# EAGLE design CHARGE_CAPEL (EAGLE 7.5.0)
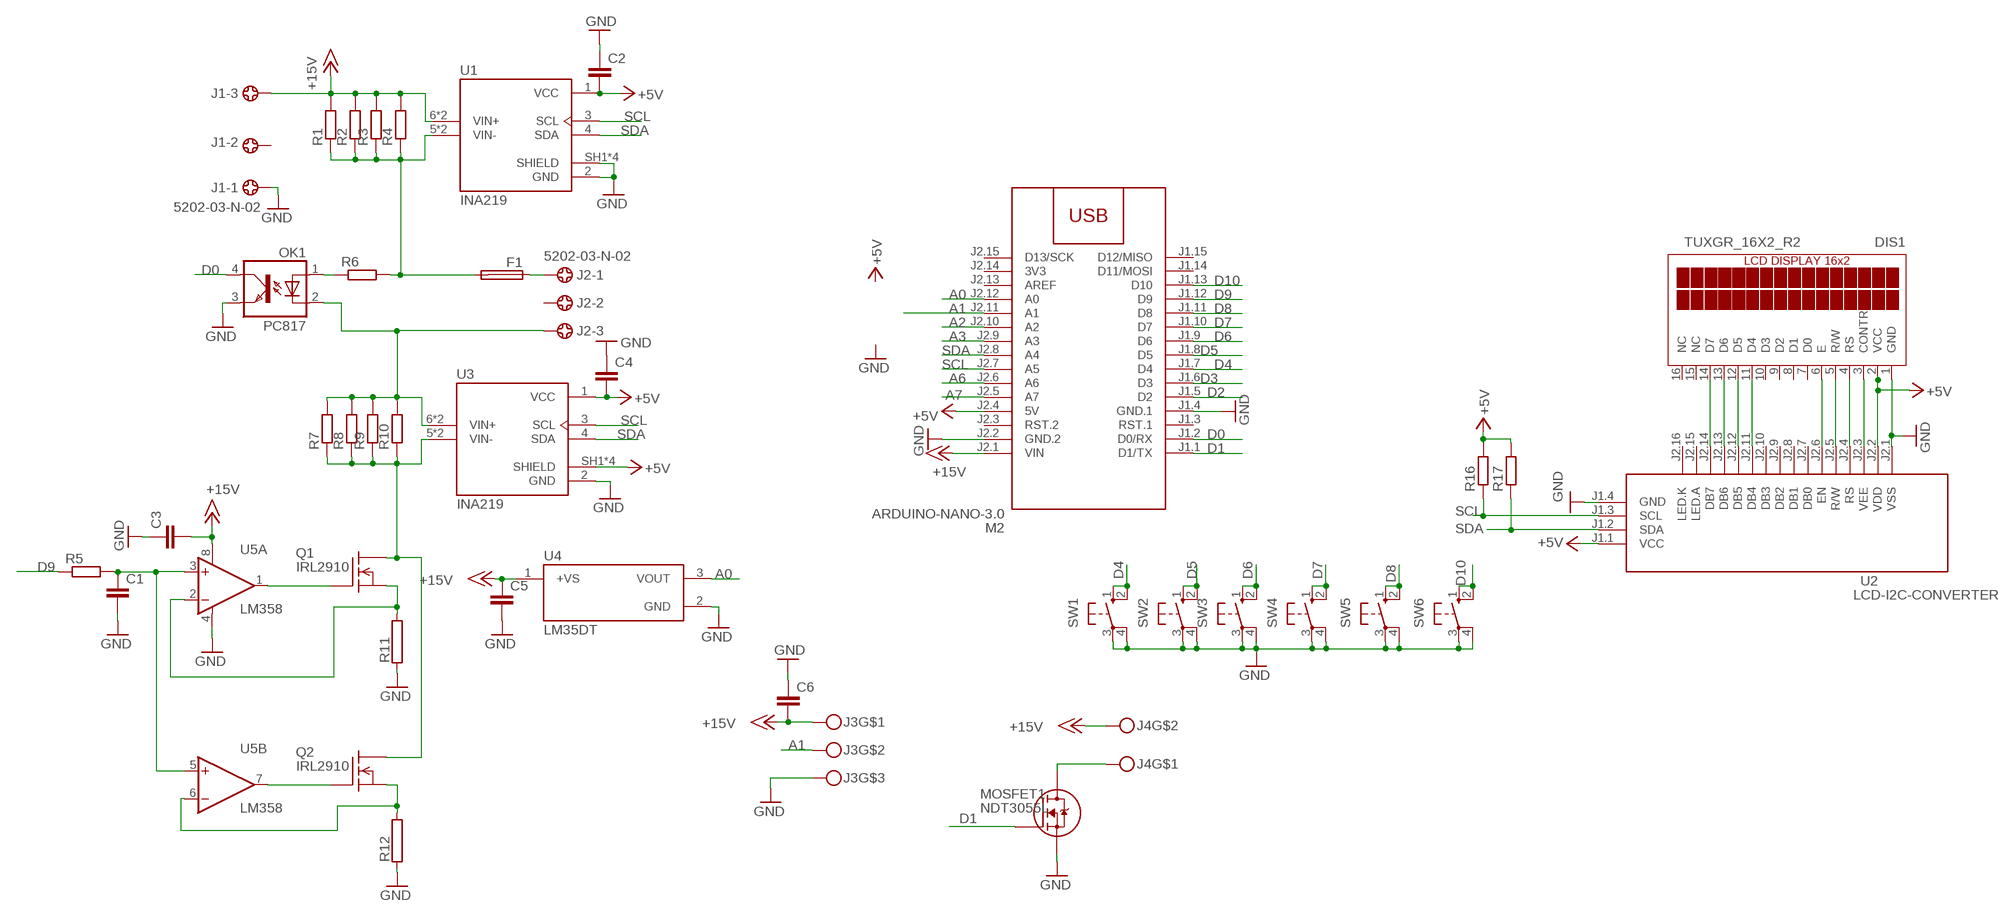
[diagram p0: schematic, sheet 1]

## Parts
C1  C-EUC1206  [C1206]
C2  C-EUC1206  [C1206]
C3  C-EUC1206  [C1206]
C4  C-EUC1206  [C1206]
C5  C-EUC1206  [C1206]
C6  C-EUC1206  [C1206]
DIS1  TUXGR_16X2_R2  [TUXGR_16X2_R2]
F1  FUSEBLANK_5X20MM  [FUSE_HOLDER_5X20MM]
J1  5202-03-N-02  [5202-03-N-02]
J2  5202-03-N-02  [5202-03-N-02]
J3  MKDSN3  [MKDSN3]
J4  MKDSN1,5-2-5,08  [MKDSN1,5-2-5,08]
M2  ARDUINO-NANO-3.0  [ARDUINO-NANO-3.0]
MOSFET1  NDT3055L  [SOT223-4]
OK1  PC817  [DIL04]
Q1  IRL2910  IRF540  [TO220]
Q2  IRL2910  IRF540  [TO220]
R1  R-EU_R2512  [R2512]
R2  R-EU_R2512  [R2512]
R3  R-EU_R2512  [R2512]
R4  R-EU_R2512  [R2512]
R5  R-EU_R1206  [R1206]
R6  R-EU_R1206  [R1206]
R7  R-EU_R2512  [R2512]
R8  R-EU_R2512  [R2512]
R9  R-EU_R2512  [R2512]
R10  R-EU_R2512  [R2512]
R11  RCA4200  [CA4200]
R12  RCA4200  [CA4200]
R16  R-EU_R1206  [R1206]
R17  R-EU_R1206  [R1206]
SW1  40-XX  [B3F-40XX]
SW2  40-XX  [B3F-40XX]
SW3  40-XX  [B3F-40XX]
SW4  40-XX  [B3F-40XX]
SW5  40-XX  [B3F-40XX]
SW6  40-XX  [B3F-40XX]
U1  INA219  [MODULE_INA219]
U2  LCD-I2C-CONVERTER  [LCD-I2C-CONVERTER]
U3  INA219  [MODULE_INA219]
U4  LM35DT  [TO254P1016X457X1955-3]
U5  LM358  OPA2234P  [DIL08]

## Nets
+5V: C2.2 C4.2 DIS1.2(VCC) M2.J2.4(5V) R16.2 R17.2 U1.1(VCC) U2.J1.1(VCC) U2.J2.2(VDD) U3.1(VCC) U3.SH1(SHIELD) U3.SH2(SHIELD) U3.SH3(SHIELD) U3.SH4(SHIELD)
+15V: C3.2 C5.1 C6.2 J1.3 J3.1 J4.2 M2.J2.1(VIN) R1.2 R2.2 R3.2 R4.2 U1.6(VIN+) U1.VIN+ U4.1(+VS) U5.8(A:V+)
A0: M2.J2.12(A0) U4.3(VOUT)
A1: J3.2 M2.J2.11(A1)
A2: M2.J2.10(A2)
A3: M2.J2.9(A3)
A6: M2.J2.6(A6)
A7: M2.J2.5(A7)
D0: M2.J1.2(D0/RX) OK1.4(COL)
D1: M2.J1.1(D1/TX) MOSFET1.1(G)
D2: M2.J1.5(D2)
D3: M2.J1.6(D3)
D4: M2.J1.7(D4) SW1.1(S) SW1.2(S1)
D5: M2.J1.8(D5) SW2.1(S) SW2.2(S1)
D6: M2.J1.9(D6) SW3.1(S) SW3.2(S1)
D7: M2.J1.10(D7) SW4.1(S) SW4.2(S1)
D8: M2.J1.11(D8) SW5.1(S) SW5.2(S1)
D9: M2.J1.12(D9) R5.1
D10: M2.J1.13(D10) SW6.1(S) SW6.2(S1)
GND: C1.2 C2.1 C3.1 C4.1 C5.2 C6.1 DIS1.1(GND) J1.1 J3.3 M2.J1.4(GND.1) M2.J2.2(GND.2) MOSFET1.3(S) OK1.3(EMIT) R11.1 R12.1 SW1.3(P) SW1.4(P1) SW2.3(P) SW2.4(P1) SW3.3(P) SW3.4(P1) SW4.3(P) SW4.4(P1) SW5.3(P) SW5.4(P1) SW6.3(P) SW6.4(P1) U1.2(GND) U1.SH1(SHIELD) U1.SH2(SHIELD) U1.SH3(SHIELD) U1.SH4(SHIELD) U2.J1.4(GND) U2.J2.1(VSS) U3.2(GND) U4.2(GND) U5.4(A:V-)
N$1: DIS1.14(D7) U2.J2.14(DB7)
N$2: DIS1.13(D6) U2.J2.13(DB6)
N$3: DIS1.12(D5) U2.J2.12(DB5)
N$4: DIS1.11(D4) U2.J2.11(DB4)
N$5: DIS1.6(E) U2.J2.6(EN)
N$6: DIS1.5(R/W) U2.J2.5(R/W)
N$7: DIS1.4(RS) U2.J2.4(RS)
N$8: Q1.1(G) U5.1(A:OUT)
N$9: F1.2 R1.1 R2.1 R3.1 R4.1 R6.2 U1.5(VIN-) U1.VIN-
N$10: DIS1.3(CONTR) U2.J2.3(VEE)
N$11: F1.1 J2.1
N$12: J2.3 OK1.2(C) R7.2 R8.2 R9.2 R10.2 U3.6(VIN+) U3.VIN+
N$13: OK1.1(A) R6.1
N$14: Q1.3(S) R11.2 U5.2(A:-IN)
N$15: Q2.3(S) R12.2 U5.6(B:-IN)
N$16: Q1.2(D) Q2.2(D) R7.1 R8.1 R9.1 R10.1 U3.5(VIN-) U3.VIN-
N$17: Q2.1(G) U5.7(B:OUT)
N$18: J4.1 MOSFET1.2(D) MOSFET1.4(D)
N$19: C1.1 R5.2 U5.3(A:+IN) U5.5(B:+IN)
SCL: M2.J2.7(A5) R16.1 U1.3(SCL) U2.J1.3(SCL) U3.3(SCL)
SDA: M2.J2.8(A4) R17.1 U1.4(SDA) U2.J1.2(SDA) U3.4(SDA)
Unconnected: DIS1.7(D0) DIS1.8(D1) DIS1.9(D2) DIS1.10(D3) DIS1.15(NC) DIS1.16(NC) J1.2 J2.2 M2.J1.3(RST.1) M2.J1.14(D11/MOSI) M2.J1.15(D12/MISO) M2.J2.3(RST.2) M2.J2.13(AREF) M2.J2.15(D13/SCK) U2.J2.7(DB0) U2.J2.8(DB1) U2.J2.9(DB2) U2.J2.10(DB3) U2.J2.15(LED.A) U2.J2.16(LED.K)

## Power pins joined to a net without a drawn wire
3V3: M2.J2.14(3V3)

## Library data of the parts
C1-C6 = rcl:C-EU: CAPACITOR, European symbol
DIS1 = display-lcd:TUXGR_16X2_R2: Tuxgraphics LCD display 16x2 characters reflective, without background light Source: tuxgr_12x2_r2.pdf; OC_FARNELL: unknown; OC_NEWARK: unknown
F1 = fuse:FUSE: Fuse; OC_FARNELL: unknown; OC_NEWARK: unknown
J1 J2 = con-ebyelectro:5202-03-N-02: Barrier Blocks Sreies 5202 Source: http://www.ebyelectro.com/PDF/5202-XX-N-02.pdf; OC_FARNELL: unknown; OC_NEWARK: unknown
J3 = con-phoenix-508:MKDSN3
J4 = con-phoenix-508:MKDSN1,5-2-5,08
M2 = diy-modules:ARDUINO-NANO-3.0: Arduino Nano 3.0 and compatible devices More details available here: https://www.arduino.cc/en/Main/ArduinoBoardNano Click here to find device on ebay.com
MOSFET1 = NDT3055L:NDT3055L: Trans MOSFET N-CH 60V 4A 4-Pin(3+Tab) SOT-223 Trans MOSFET N-CH 60V 4A 4-Pin(3+Tab) SOT-223 Check availability; AVAILABILITY: In Stock; CHECK_PRICES: https://www.snapeda.com/parts/NDT3055L/Onsemi/view-part/?ref=eda; DESCRIPTION: Trans MOSFET N-CH 60V 4A 4-Pin(3+Tab) SOT-223 Trans MOSFET N-CH 60V 4A 4-Pin(3+Tab) SOT-223; MF: ON; MP: NDT3055L; PACKAGE: SOT-223-4 Fairchild Semiconductor; PRICE: None; SNAPEDA_LINK: https://www.snapeda.com/parts/NDT3055L/Onsemi/view-part/?ref=snap
OK1 = optocoupler:PC817: SHARP OPTO COUPLER; MPN: PC817X4J000F; OC_FARNELL: 9707727; OC_NEWARK: 97K7059
Q1 Q2 = transistor-fet:IRF540: N-Channel Enhancement MOSFET (HEXFET); 100V; 28A; 0,077Ohm
R1-R10 R16 R17 = rcl:R-EU_: RESISTOR, European symbol
R11 R12 = resistor-power:R: Power Resitor; OC_FARNELL: unknown; OC_NEWARK: unknown
SW1-SW6 = switch-omron:40-XX: OMRON SWITCH; MF: OMRON COMPONENTS USA; MPN: B3F-4000; OC_FARNELL: 176434; OC_NEWARK: 36K3105
U1 U3 = INA219:INA219: Check availability; AVAILABILITY: Not in stock; CHECK_PRICES: https://www.snapeda.com/parts/INA219%20High%20Side%20DC%20Current%20Sensor%20Breakout%20-%2026V%20%C2%B13.2A%20Max%20-%20STEMMA%20QT/Adafruit+Industries/view-part/?ref=eda; DESCRIPTION: INA219 High Side DC Current Sensor Breakout - 26V ±3.2A Max | Adafruit Industries 904; MF: Adafruit Industries; MP: INA219 High Side DC Current Sensor Breakout - 26V ±3.2A Max - STEMMA QT; PACKAGE: NON-STANDARD-8 ADAFRUIT; PRICE: None; SNAPEDA_LINK: https://www.snapeda.com/parts/INA219%20High%20Side%20DC%20Current%20Sensor%20Breakout%20-%2026V%20%C2%B13.2A%20Max%20-%20STEMMA%20QT/Adafruit+Industries/view-part/?ref=snap
U2 = diy-modules:LCD-I2C-CONVERTER: I2C Bus to 4-Bit Parallel LCD Interface with LED backlight driver
U4 = LM35DT-H:LM35DT: Check availability; AVAILABILITY: In Stock; CHECK_PRICES: https://www.snapeda.com/parts/LM35DT/Texas+Instruments/view-part/?ref=eda; DESCRIPTION: ±0.5°C 4V-30V, Temperature sensor with analog output 3-TO-220 0 to 100; MF: Texas Instruments; MP: LM35DT; PACKAGE: TO-220-3 Texas Instruments; PRICE: None; SNAPEDA_LINK: https://www.snapeda.com/parts/LM35DT/Texas+Instruments/view-part/?ref=snap
U5 = burr-brown:OPA2234: Operational Amplifier; OC_FARNELL: unknown; OC_NEWARK: unknown

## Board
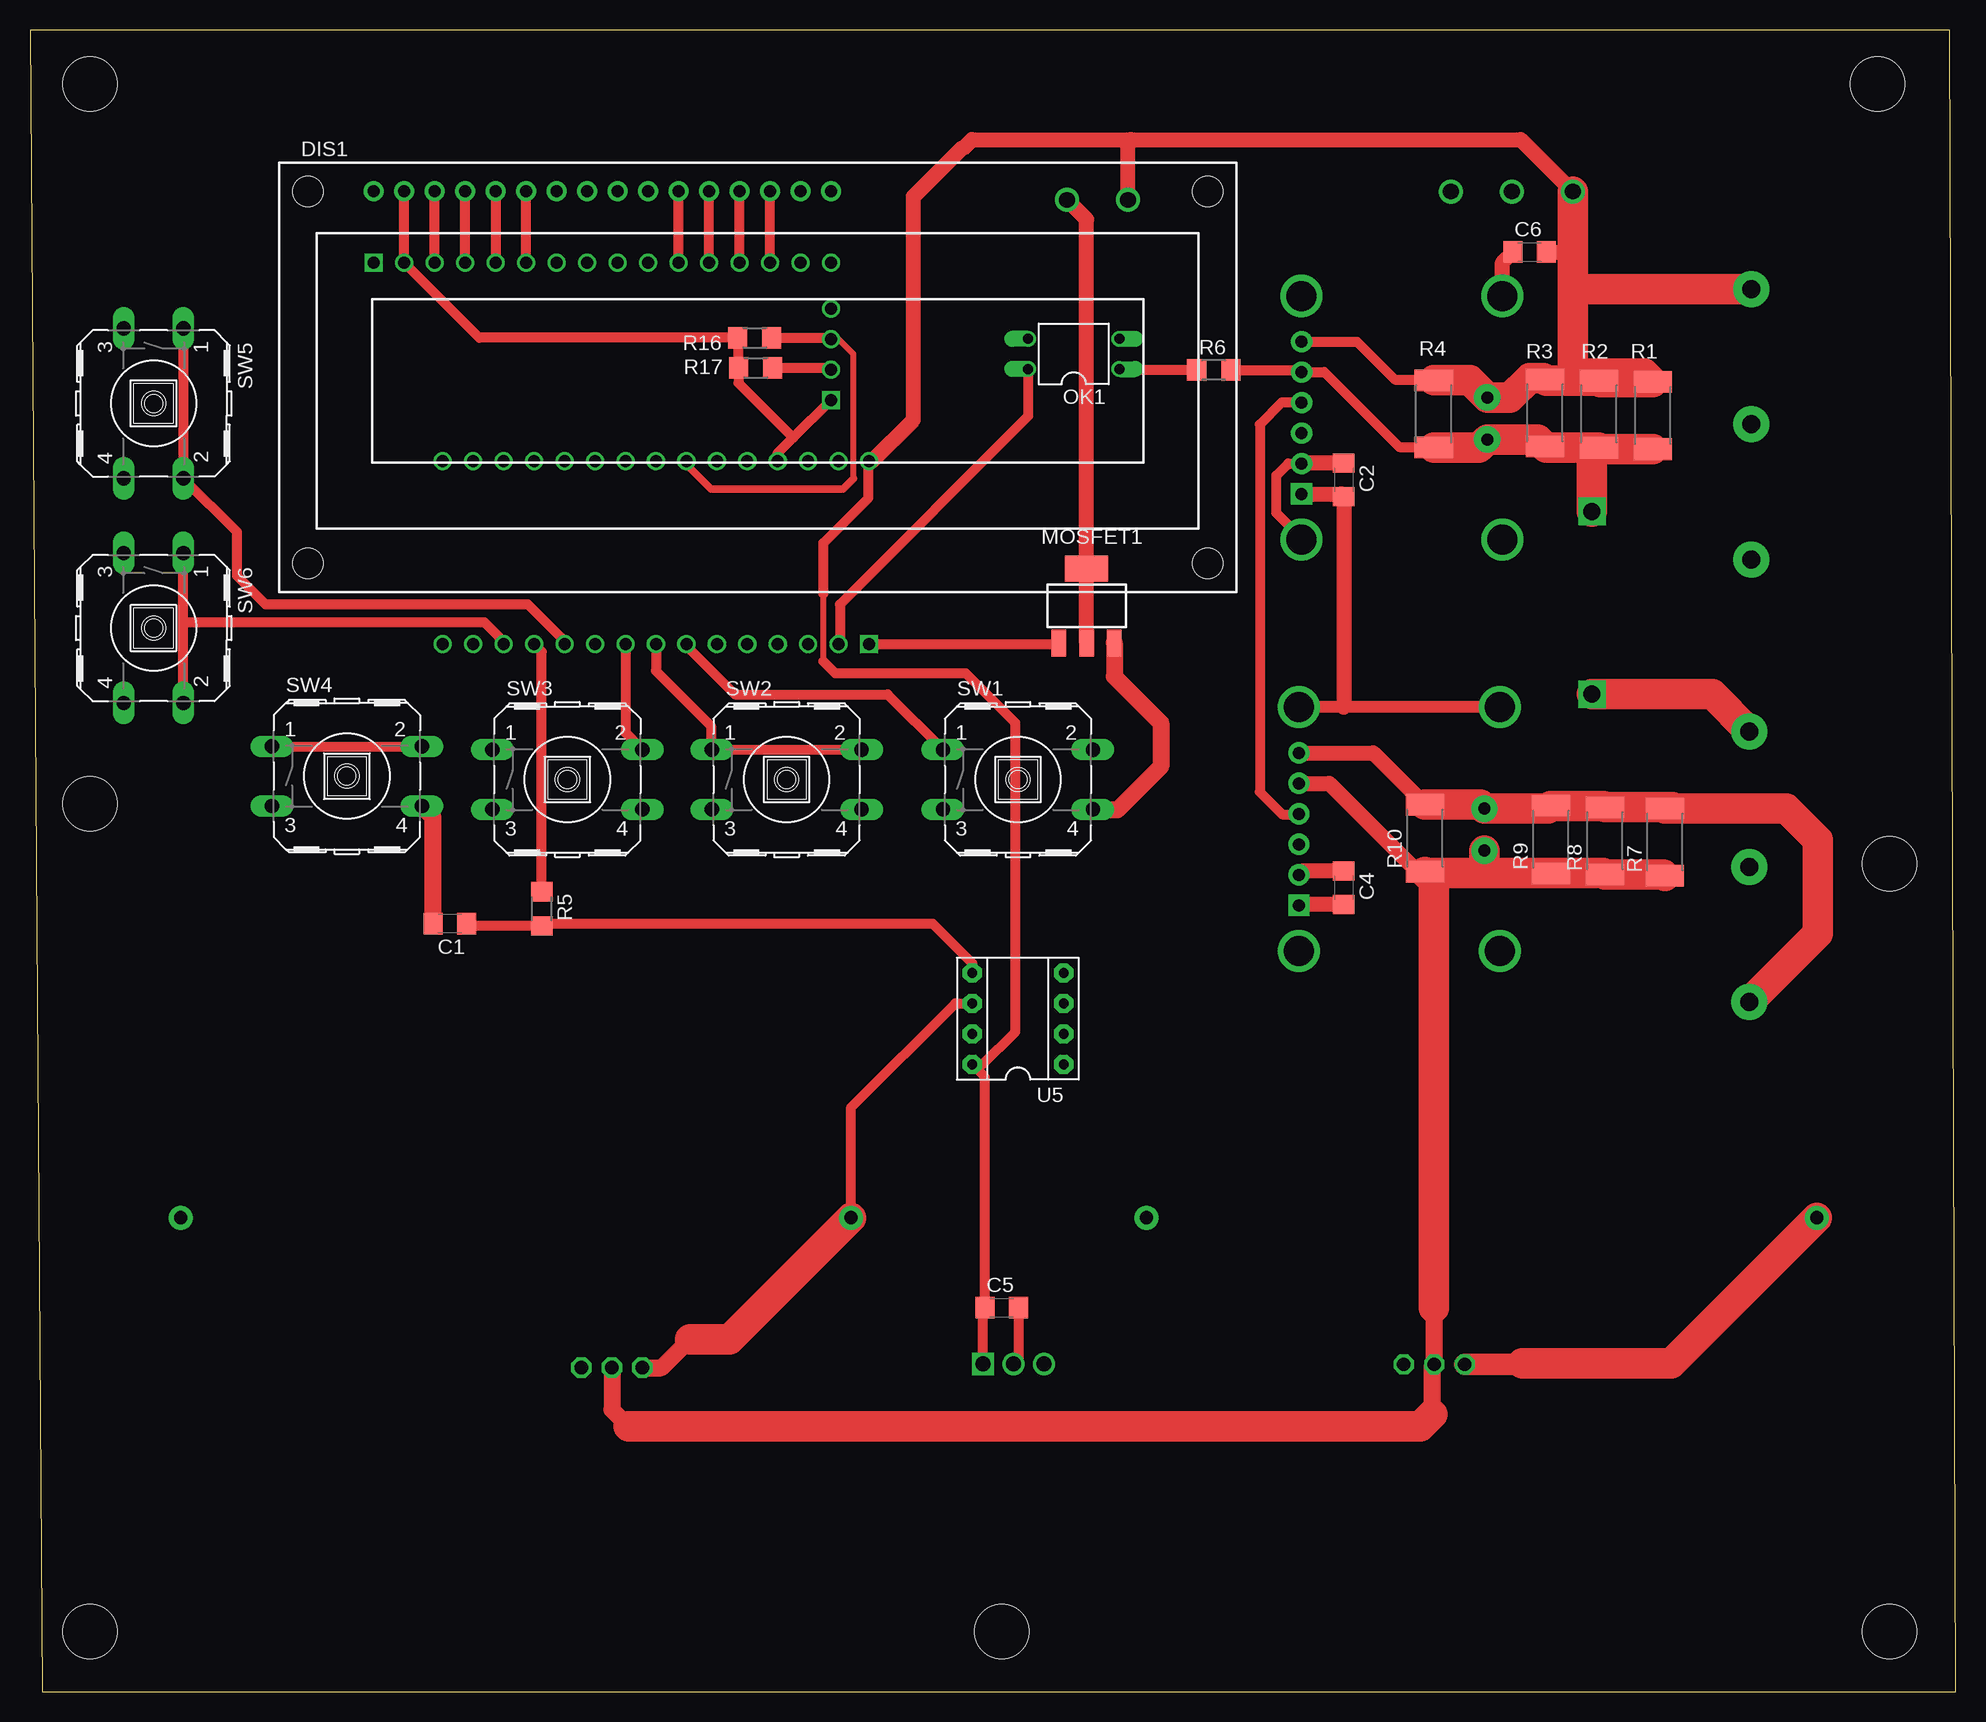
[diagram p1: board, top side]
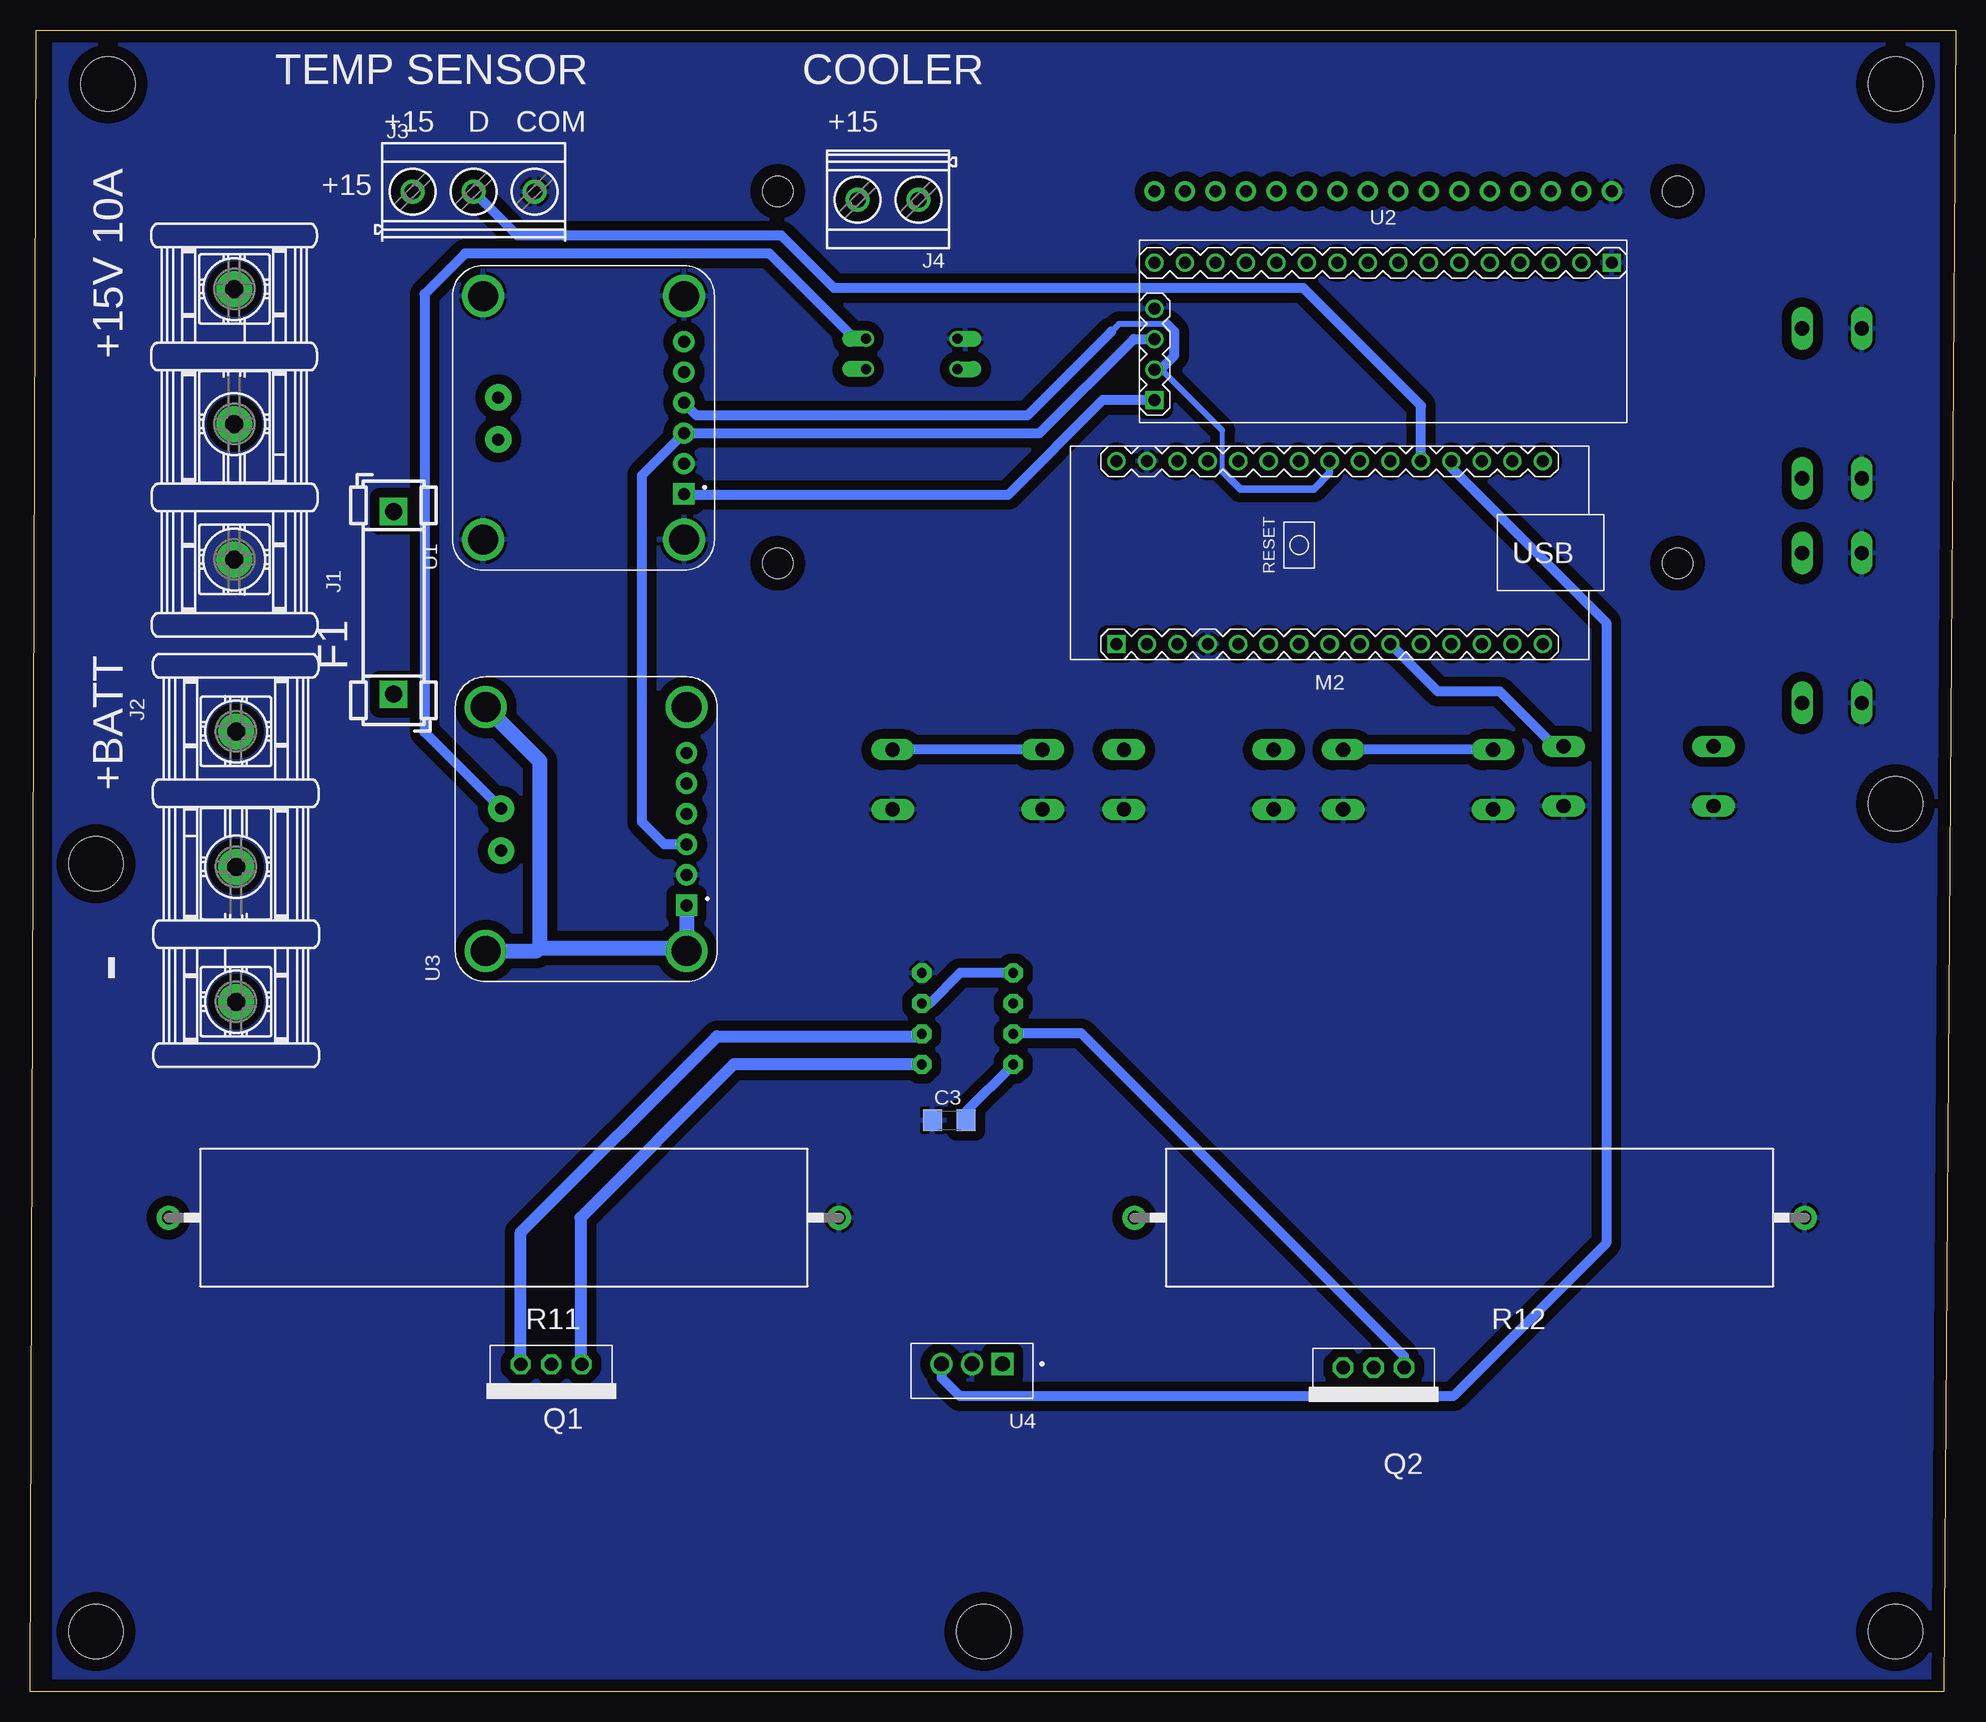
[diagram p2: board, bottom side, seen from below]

Size 160.5 x 138.5 mm. Coordinates in mm from the lower left corner, seen from the top.
Outline: 1,0 160.5,0 160,138.5 0,138.5 1,0
Copper layers (1*16): Top 0.035mm / dielectric 1.5mm / Bottom 0.035mm
Design rules "default": minimum track width 10mil, minimum drill 24mil, track to track 8mil, track to pad 8mil, pad to pad 8mil, via to via 8mil, smd to smd 8mil, copper to edge 40mil, drill to drill 8mil, minimum pad ring 10mil, minimum via ring 8mil, stop-mask expansion 4mil, vias tented up to drill 0mil, thermal gap 10mil
Holes 4.5 mm at 5,134 5,74 5,5 81,5 155,5 155,69 154,134

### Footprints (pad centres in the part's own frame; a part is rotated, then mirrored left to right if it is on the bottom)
C1206 = smd 1.6 x 1.8: 1 -1.4,0; 2 1.4,0
TUXGR_16X2_R2 = drill 1 pad 1.676: 1 -32,15.5; 2 -29.46,15.5; 3 -26.92,15.5; 4 -24.38,15.5; 5 -21.84,15.5; 6 -19.3,15.5; 7 -16.76,15.5; 8 -14.22,15.5; 9 -11.68,15.5; 10 -9.14,15.5; 11 -6.6,15.5; 12 -4.06,15.5; 13 -1.52,15.5; 14 1.02,15.5; 15 3.56,15.5; 16 6.1,15.5 | hole 2.5: -37.5,-15.5; 37.5,-15.5; -37.5,15.5; 37.5,15.5
FUSE_HOLDER_5X20MM = drill 1.422 pad 2.286 square: 1 0,0; 2 15.24,0
5202-03-N-02 = drill 1.5 pad 3: 1 -9.29,0; 2 2,0; 3 13.25,0
MKDSN3 = drill 1.3 pad 2: 1 -5.101,0.025; 2 -0.021,0.025; 3 5.059,0.025
MKDSN1,5-2-5,08 = drill 1.3 pad 2: 1 -2.561,0.025; 2 2.519,0.025
ARDUINO-NANO-3.0 = drill 1 square: J1.1 17.78,7.62 | drill 1: J1.2 15.24,7.62; J1.3 12.7,7.62; J1.4 10.16,7.62; J1.5 7.62,7.62; J1.6 5.08,7.62; J1.7 2.54,7.62; J1.8 0,7.62; J1.9 -2.54,7.62; J1.10 -5.08,7.62; J1.11 -7.62,7.62; J1.12 -10.16,7.62; J1.13 -12.7,7.62; J1.14 -15.24,7.62; J1.15 -17.78,7.62; J2.1 17.78,-7.62; J2.2 15.24,-7.62; J2.3 12.7,-7.62; J2.4 10.16,-7.62; J2.5 7.62,-7.62; J2.6 5.08,-7.62; J2.7 2.54,-7.62; J2.8 0,-7.62; J2.9 -2.54,-7.62; J2.10 -5.08,-7.62; J2.11 -7.62,-7.62; J2.12 -10.16,-7.62; J2.13 -12.7,-7.62; J2.14 -15.24,-7.62; J2.15 -17.78,-7.62
SOT223-4 = smd 1.219 x 2.235: 1 -2.24,-3.091; 2 0.071,-3.091; 3 2.383,-3.091 | smd 3.6 x 2.2: 4 0.071,3.107
DIL04 = drill 0.813 offset: 1 -1.27,-3.81; 2 1.27,-3.81; 3 1.27,3.81; 4 -1.27,3.81
TO220 = drill 1.118 octagon: 1 -2.54,0; 2 0,0; 3 2.54,0
R2512 = smd 1.8 x 3.2: 1 -2.8,0; 2 2.8,0
R1206 = smd 1.6 x 1.803: 1 -1.422,0; 2 1.422,0
CA4200 = drill 1.1 pad 2: 1 -27.94,0; 2 27.94,0
B3F-40XX = drill 1.194 long: 1 -6.248,2.489; 2 6.248,2.489; 3 -6.248,-2.489; 4 6.248,-2.489
MODULE_INA219 = drill 1 pad 1.778 square: 1 -6.35,-9.12 | drill 1 pad 1.778: 2 -3.81,-9.12; 3 -1.27,-9.12; 4 1.27,-9.12; 5 3.81,-9.12; 6 6.35,-9.12 | drill 2.5 pad 3.2: SH1 -10.16,7.62; SH2 10.16,7.62; SH3 -10.16,-9.12; SH4 10.16,-9.12 | drill 1 pad 2.184: VIN+ 1.7,6.35; VIN- -1.8,6.35
LCD-I2C-CONVERTER = drill 1 square: J1.1 -19.05,-5.08; J2.1 19.05,6.35 | drill 1: J1.2 -19.05,-2.54; J1.3 -19.05,0; J1.4 -19.05,2.54; J2.2 16.51,6.35; J2.3 13.97,6.35; J2.4 11.43,6.35; J2.5 8.89,6.35; J2.6 6.35,6.35; J2.7 3.81,6.35; J2.8 1.27,6.35; J2.9 -1.27,6.35; J2.10 -3.81,6.35; J2.11 -6.35,6.35; J2.12 -8.89,6.35; J2.13 -11.43,6.35; J2.14 -13.97,6.35; J2.15 -16.51,6.35; J2.16 -19.05,6.35
TO254P1016X457X1955-3 = drill 1.24 square: 1 -2.54,-0.573 | drill 1.24: 2 0,-0.573; 3 2.54,-0.573
DIL08 = drill 0.813 pad 1.6 octagon: 1 -3.81,-3.81; 2 -1.27,-3.81; 3 1.27,-3.81; 4 3.81,-3.81; 5 3.81,3.81; 6 1.27,3.81; 7 -1.27,3.81; 8 -3.81,3.81

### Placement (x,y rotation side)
C1  35,64 180 top
C2  109.5,101 270 top
C3  83.88,47.62 0 bottom
C4  109.5,67 270 top
C5  81,32 0 top
C6  125,120 0 top
DIS1  60.66,109.55 0 top
F1  130.2,83.13 90 bottom
J1  143.47,103.66 90 bottom
J2  143.33,70.75 270 bottom
J3  123.5,125 0 bottom
J4  89,124.38 180 bottom
M2  52.17,94.93 180 bottom
MOSFET1  88,90.5 0 top
OK1  87,111.5 90 top
Q1  117.05,27.27 180 bottom
Q2  48.5,27 180 bottom
R1  135.27,106.36 90 top
R2  130.77,106.47 90 top
R3  126.27,106.58 90 top
R4  117,106.5 90 top
R5  42.66,65.24 270 top
R6  98.68,110.16 0 top
R7  136.27,70.8 90 top
R8  131.27,70.91 90 top
R9  126.77,71.02 90 top
R10  116.27,71.13 90 top
R11  121,39.5 180 bottom
R12  40.5,39.5 180 bottom
R16  60.4,112.84 180 top
R17  60.48,110.34 180 top
SW1  82.35,76.02 0 top
SW2  63.07,76.02 0 top
SW3  44.79,76.02 0 top
SW4  26.41,76.3 0 top
SW5  10.3,107.37 270 top
SW6  10.3,88.65 270 top
U1  115.11,106.17 90 bottom
U2  47.71,112.74 0 bottom
U3  114.89,71.89 90 bottom
U4  81.98,26.73 180 bottom
U5  82.35,56.09 90 top

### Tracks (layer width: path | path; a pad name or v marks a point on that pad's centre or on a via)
+5V
  Top 0.813: M2.J2.4 62.33,103.23 63.61,104.51 | 63.61,104.51 U2.J1.1 | 63.61,104.51 59.06,109.07 R17.2 59.06,112.76 R16.2 37.45,112.84 U2.J2.2 DIS1.2
  Top 1.016: U3.SH2 109.5,82.05 U3.SH4
  Top 1.27: C4.2 105.83,65.6 U3.1 | 109.5,82.05 C2.2 109.28,99.82 U1.1
  Bottom 0.813: U2.J1.1 71.09,107.66 79,99.75 105.92,99.75 U1.1
  Bottom 1.27: U3.1 U3.SH3 106.04,62 118,62 | U3.SH1 118.27,61.73 118,62 | 118,62 118,77.54 U3.SH2
+15V
  Top 0.5: 66.12,85.88 66.12,91.5
  Top 0.813: U1.6 110.61,112.52 113.75,109.38 116.92,109.38 R4.2 | 66.12,85.88 67.12,84.88 78,84.88 82.12,80.75 82.12,55 79.41,52.28 U5.8 79.6,51.22 C5.1 79.44,31.84 U4.1 | 66.12,91.5 66.12,95.75 69.88,99.5 69.88,102.47 M2.J2.1
  Top 1.27: C6.2 128.48,120 128.6,119.88 | M2.J2.1 70.17,102.55 73.62,106 73.62,124.62 77.62,128.62 77.75,128.62 78.5,129.38 91.75,129.38 | 91.75,129.38 124.25,129.38 J3.1 | J4.2 91.52,129.14 91.75,129.38
  Top 2.54: R4.2 120.03,109.3 U1.VIN+ 123.37,107.87 125,109.5 126.15,109.5 R3.2 126.38,109.27 R2.2 130.88,109.16 R1.2 134.56,109.88 128.75,109.88 128.6,110.02 128.6,117.12 | J3.1 128.6,119.88 128.6,117.12 | J1.3 128.82,116.91 128.6,117.12
  Bottom 0.813: C3.2 82.47,48.34 U5.8
A0
  Bottom 0.813: M2.J2.12 42.01,102.01 29.12,89.12 29.12,37.38 41.88,24.62 83,24.62 84.5,26.12 84.5,27.28 U4.3
A1
  Bottom 0.813: M2.J2.11 44.55,107.17 54.38,117 93.5,117 97.88,121.38 119.87,121.38 J3.2
D0
  Top 0.813: OK1.4 83.19,106.31 67.5,90.62 67.5,87.4 M2.J1.2
D1
  Top 0.813: M2.J1.1 85.66,87.31 MOSFET1.1
D4
  Top 0.813: M2.J1.7 54.71,87.17 58.75,83.12 71.49,83.12 SW1.1
  Bottom 0.813: SW1.1 SW1.2
D5
  Top 0.813: M2.J1.8 52.17,85.08 56.75,80.5 56.75,78.58 SW2.1 SW2.2
D6
  Top 0.813: M2.J1.9 49.63,79.92 SW3.2
  Bottom 0.813: SW3.1 SW3.2
D7
  Top 0.813: SW4.1 SW4.2
  Bottom 0.813: SW4.2 33.41,78.79 38,83.38 43.16,83.38 M2.J1.10
D8
  Top 0.813: SW5.1 SW5.2 17.25,96.66 17.25,93 19.62,90.62 41.5,90.62 44.55,87.58 M2.J1.11
D9
  Top 0.813: R5.1 42.66,86.66 M2.J1.12
D10
  Top 0.813: SW6.2 12.79,89.12 | 12.79,89.12 SW6.1 | M2.J1.13 39.47,87.53 37.88,89.12 12.79,89.12
GND
  Top 0.813: U1.SH3 105.99,96.14 103.88,98.25 103.88,101.38 104.88,102.38 105.97,102.38 U1.2 | C5.2 82.4,27.72 U4.2
  Top 1.27: C4.1 106.09,68.4 U3.2 | C2.1 106.03,102.4 U1.2 | U1.SH2 122.73,119.13 C6.1
  Top 1.422: MOSFET1.3 90.38,84.62 94.25,80.75 94.25,77.12 90.62,73.5 88.63,73.5 SW1.4 | C1.2 33.6,72.87 SW4.4
  pour Bottom (isolate 0.813): 1.5,137.5 158.5,137.5 158.5,0 1.5,0
N$1
  Top 0.813: U2.J2.14 DIS1.14
N$2
  Top 0.813: U2.J2.13 DIS1.13
N$3
  Top 0.813: U2.J2.12 DIS1.12
N$4
  Top 0.813: U2.J2.11 DIS1.11
N$5
  Top 0.813: U2.J2.6 DIS1.6
N$6
  Top 0.813: DIS1.5 U2.J2.5
N$7
  Top 0.813: U2.J2.4 DIS1.4
N$8
  Bottom 1.016: U5.1 101.84,52.28 114.62,39.5 114.62,27.39 Q1.1
N$9
  Top 0.813: R6.2 105.81,110.16 U1.5 107.89,109.98 114.12,103.75 116.95,103.75 R4.1
  Top 2.54: R1.1 130.88,103.56 R2.1 | R2.1 126.38,103.67 R3.1 125.68,104.37 U1.VIN- 120.79,103.7 R4.1 | F1.2 130.2,103.1 R2.1
N$10
  Top 0.813: U2.J2.3 DIS1.3
N$11
  Top 2.54: F1.1 140.24,83.13 J2.1
N$12
  Top 1.27: U3.6 111.96,78.24 R10.2
  Top 2.54: R7.2 137,73.6 | 137,73.6 146.4,73.6 149,71 149,63.17 J2.3 | 137,73.6 136.89,73.71 R8.2 131.16,73.82 R9.2 126.54,73.59 U3.VIN+ 120.9,73.93 R10.2
  Bottom 0.5: 126.62,78.97 U3.VIN+
  Bottom 0.813: OK1.2 91.77,112.77 98.88,119.88 124.25,119.88 127.62,116.5 127.62,79.97 U3.VIN+
N$13
  Top 0.813: R6.1 90.88,110.16 OK1.1
N$14
  Top 1.778: Q1.3 124.27,27.27 124.38,27.38
  Top 2.54: 124.38,27.38 136.81,27.38 R11.2
  Bottom 1.016: Q1.3 119.59,38.28 103.25,54.62 86.36,54.62 U5.2
N$15
  Top 0.813: R12.2 68.44,48.69 77.12,57.38 78.53,57.38 U5.6
  Top 1.422: Q2.3 52.62,27 55,29.38
  Top 2.54: 55,29.38 58.31,29.38 R12.2
N$16
  Top 1.27: U3.5 108.3,75.7 115.5,68.5 116.1,68.5 R10.1
  Top 1.422: 117,32 117.05,31.95 Q1.2 116.88,27.09 116.88,23.12 | Q2.2 48.5,23.5 49.88,22.12
  Top 2.54: 121.5,68.22 R9.1 131.16,68.22 R8.1 136.16,68.11 R7.1 | 121.5,68.22 116.38,68.22 R10.1 117,67.6 117,32 | U3.VIN- 121.24,68.48 121.5,68.22 | 49.88,22.12 115.88,22.12 116.88,23.12
N$17
  Bottom 0.813: Q2.1 45.96,27.96 72.88,54.88 78.48,54.88 U5.7
N$18
  Top 1.27: J4.1 88.07,122.72 MOSFET1.4 MOSFET1.2
N$19
  Top 0.813: U5.5 78.54,60.71 75.25,64 42.84,64 R5.2 36.58,63.82 C1.1
  Bottom 0.813: U5.5 82.97,59.9 85.5,57.38 86.14,57.38 U5.3
SCL
  Top 0.5: 68.62,101.12 68.62,111.5 67.38,112.75 U2.J1.3
  Top 0.61: M2.J2.7 54.71,102.29 56.75,100.25 67.75,100.25 68.62,101.12
  Top 0.813: R16.1 66.66,112.84 U2.J1.3
  Bottom 0.813: U3.3 107.62,70.62 109.5,72.5 109.5,101.39 U1.3 76.35,104.9 68.5,112.75 U2.J1.3
SDA
  Top 0.813: U1.4 104.31,107.44 102.5,105.62 102.5,75 104.38,73.12 105.73,73.12 U3.4 | R17.1 66.62,110.34 U2.J1.2
  Bottom 0.406: 61.12,101.75 61.12,105.12
  Bottom 0.5: 65.75,114 69.75,114 70.38,113.38 | 61.12,105.12 66.25,110.25
  Bottom 0.61: M2.J2.8 52.17,101.58 53.5,100.25 59.62,100.25 61.12,101.75
  Bottom 0.813: U2.J1.2 66.3,110.2 66.25,110.25 65.12,111.38 65.12,113.38 65.75,114 | 70.38,113.38 77.38,106.38 104.92,106.38 U1.4

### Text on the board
bNames: COOLER | TEMP SENSOR | +15 | COM | D | +15 | +15 | +15V 10A | +BATT | -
